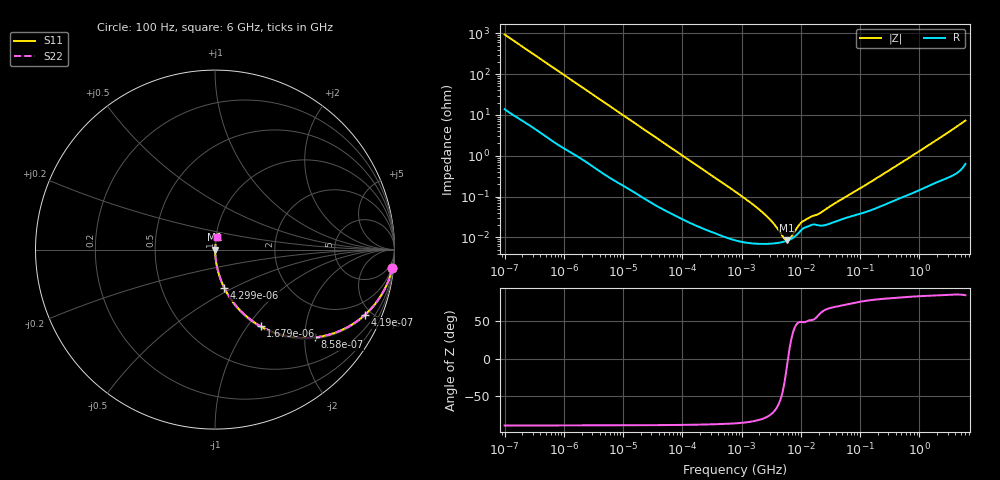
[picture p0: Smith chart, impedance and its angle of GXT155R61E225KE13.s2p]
!Murata Part Number: GXT155R61E225KE13
!These Parameters are Measured in Series Mode Connection
!Data Generated on Jan 08, 2026
!  o--ll--o
!Port1  Port2
!  o------o
!Operation Temp=25[degC], DC Bias Voltage=0[V]
!Freq. Start=100[Hz] Stop=6[GHz] 401[Steps]
# Hz S RI R 50
!Freq.(Hz) S11(Real) S11(Imag) S21(Real) S21(Imag) S12(Real) S12(Imag) S22(Real) S22(Imag)
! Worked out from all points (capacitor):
!   401 points, 100 Hz to 6 GHz, reference 50 ohm
!   read as one part in series: C = 1.68 uF near 109 Hz
!   lowest |Z| = 8.37 mohm at 5.809 MHz (marker M1)
!   series resonance near 6.081 MHz, so ESL is about 410 pH
!   S11 on the Smith chart (normalised r, x): 100 Hz: 1, -19; 419 Hz: 1.07, -4.57; 858 Hz: 1.03, -2.24; 1.679 kHz: 1.02, -1.15; 4.299 kHz: 1.01, -0.46; 6 GHz: 1.01, +0.14
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100  0.9874 -0.1044  0.0126 0.1044  0.0126 0.1044  0.9874 -0.1044
224  0.9444 -0.2216  0.0556 0.2216  0.0556 0.2216  0.9444 -0.2216
419  0.8352 -0.3633  0.1648 0.3633  0.1648 0.3633  0.8352 -0.3633
858  0.5567 -0.4891  0.4433 0.4891  0.4433 0.4891  0.5567 -0.4891
1174  0.4053 -0.483  0.5947 0.483  0.5947 0.483  0.4053 -0.483
1679  0.2536 -0.4268  0.7464 0.4268  0.7464 0.4268  0.2536 -0.4268
2008  0.1937 -0.3868  0.8063 0.3868  0.8063 0.3868  0.1937 -0.3868
4299  0.0527 -0.215  0.9473 0.215  0.9473 0.215  0.0527 -0.215
11009  0.00967 -0.0888  0.9903 0.0888  0.9903 0.0888  0.00967 -0.0888
40335  0.00117 -0.0249  0.9988 0.0249  0.9988 0.0249  0.00117 -0.0249
774597  8.61e-05 -0.00133  0.9999 0.00133  0.9999 0.00133  8.61e-05 -0.00133
2268635  6.89e-05 -0.000401  0.9999 0.000401  0.9999 0.000401  6.89e-05 -0.000401
3394479  7.04e-05 -0.000215  0.9999 0.000215  0.9999 0.000215  7.04e-05 -0.000215
4856642  7.61e-05 -7.95e-05  0.9999 7.95e-05  0.9999 7.95e-05  7.61e-05 -7.95e-05
5809218  8.21e-05 -1.6e-05  0.9999 1.6e-05  0.9999 1.6e-05  8.21e-05 -1.6e-05
6948629  9.22e-05 4.73e-05  0.9999 -4.73e-05  0.9999 -4.73e-05  9.22e-05 4.73e-05
1.039699e7  0.000155 0.000178  0.9998 -0.000178  0.9998 -0.000178  0.000155 0.000178
1.555665e7  0.000203 0.000259  0.9998 -0.000259  0.9998 -0.000259  0.000203 0.000259
2.128304e7  0.000194 0.000345  0.9998 -0.000345  0.9998 -0.000345  0.000194 0.000345
3.124326e8  0.000726 0.00436  0.9993 -0.00436  0.9993 -0.00436  0.000726 0.00436
1.873145e9  0.00269 0.0231  0.9973 -0.0231  0.9973 -0.0231  0.00269 0.0231
6e9  0.0114 0.0712  0.9886 -0.0712  0.9886 -0.0712  0.0114 0.0712
